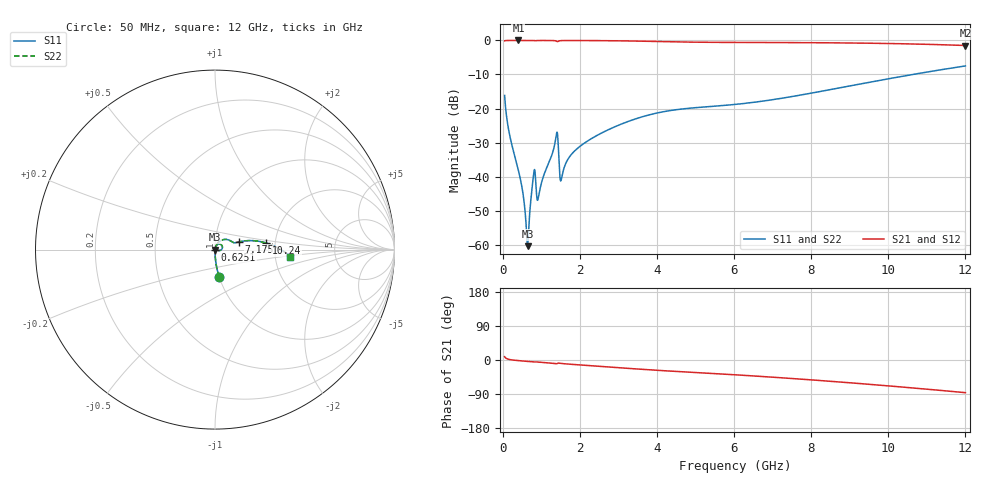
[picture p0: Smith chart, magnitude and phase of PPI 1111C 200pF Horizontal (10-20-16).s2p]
# MHz S MA R 50
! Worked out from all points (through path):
!   1601 points, 50 MHz to 12 GHz, reference 50 ohm
!   highest |S21| = -0.01 dB at 408.5 MHz (marker M1); lowest = -1.5 dB at 12 GHz (marker M2)
!   group delay of S21, straight-line fit = 19.4 ps
!   lowest |S11| = -60.5 dB at 647.5 MHz (marker M3), VSWR 1.00, Z = 50.1 + j0.000346 ohm
!   |S11| at or under -10 dB: start of sweep to 10.64 GHz
!   |S22| runs from -60.5 to -7.5 dB; largest |S21 - S12| = 0
!   S11 on the Smith chart (normalised r, x): 50 MHz: 1.00, -0.31; 625.1 MHz: 1.00, -0.00; 7.175 GHz: 1.30, +0.11; 10.24 GHz: 1.79, +0.14; 12 GHz: 2.43, -0.23
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50  0.1555 -81.2  0.9876 8.7  0.9876 8.7  0.1555 -81.2
184.4375  0.03972 -88.1  0.9987 1.2  0.9987 1.2  0.03972 -88.1
408.5  0.01226 -88.6  0.9993 -1.6  0.9993 -1.6  0.01226 -88.6
520.5312  0.00593 -85.5  0.9992 -2.6  0.9992 -2.6  0.00593 -85.5
625.0938  0.001312 -50.9  0.9991 -3.5  0.9991 -3.5  0.001312 -50.9
647.5  0.0009494 0.2  0.999 -3.7  0.999 -3.7  0.0009494 0.2
684.8438  0.002148 55.1  0.9989 -4.0  0.9989 -4.0  0.002148 55.1
759.5312  0.00657 65.3  0.9977 -4.7  0.9977 -4.7  0.00657 65.3
796.875  0.01024 55.1  0.9948 -5.1  0.9948 -5.1  0.01024 55.1
938.7812  0.005378 57.8  0.9975 -5.7  0.9975 -5.7  0.005378 57.8
1371.969  0.03507 59.6  0.987 -9.7  0.987 -9.7  0.03507 59.6
1409.312  0.0449 29.1  0.9645 -9.7  0.9645 -9.7  0.0449 29.1
1528.812  0.009515 48.5  0.9948 -9.2  0.9948 -9.2  0.009515 48.5
1723  0.01914 71.3  0.9971 -10.9  0.9971 -10.9  0.01914 71.3
2044.156  0.02893 70.6  0.9964 -13.3  0.9964 -13.3  0.02893 70.6
4038.312  0.08674 40.4  0.9638 -27.4  0.9638 -27.4  0.08674 40.4
6025  0.1148 19.3  0.9345 -39.0  0.9345 -39.0  0.1148 19.3
7175.188  0.1396 17.8  0.9311 -46.5  0.9311 -46.5  0.1396 17.8
8019.156  0.1688 16.5  0.9268 -52.6  0.9268 -52.6  0.1688 16.5
10013.31  0.2738 8.5  0.9012 -68.4  0.9012 -68.4  0.2738 8.5
10237.38  0.2886 7.2  0.8965 -70.3  0.8965 -70.3  0.2886 7.2
12000  0.422 -5.2  0.8422 -86.2  0.8422 -86.2  0.422 -5.2
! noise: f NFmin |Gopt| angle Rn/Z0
50  0.0003693  0.8651  0.3818  0.0005877
1372  0.01263  0.8907  7.84  0.02505
2701  0.01337  0.8078  15.31  0.01422
4031  0.035  0.8878  22.71  0.06516
5360  0.05358  0.9041  29.88  0.1144
6682  0.06082  0.8982  36.76  0.1177
8012  0.06537  0.8909  43.38  0.1127
9341  0.0702  0.8865  49.69  0.1107
1.067e+04  0.07586  0.8852  55.69  0.1122
1.2e+04  0.08252  0.8866  61.36  0.117
